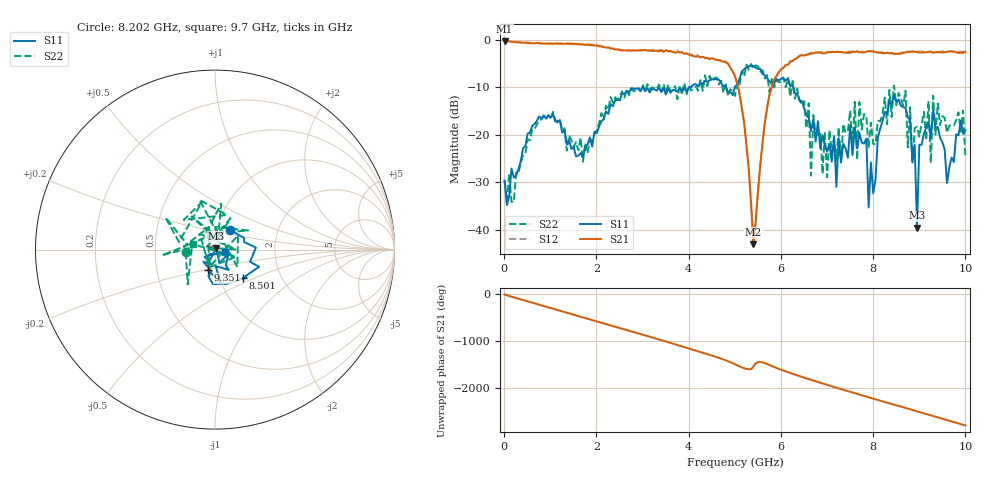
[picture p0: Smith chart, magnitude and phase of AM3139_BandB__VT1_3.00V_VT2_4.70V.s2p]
! Date/Time: Tue, Nov 13, 2018 5:00 PM
! Network Analyzer: Agilent Technologies E8364B Rev: A.07.50.67
! Sweep from 0.010 to 10.000 GHz, 201 Points, Sweep Type: LIN
! Power Supply: 3.001 V, 0.000 A
# Hz S DB R 50
!freq MagS11 AngS11 MagS21 AngS21 MagS12 AngS12 MagS22 AngS22
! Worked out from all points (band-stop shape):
!   201 points, 10 MHz to 10 GHz, reference 50 ohm
!   highest |S21| = -0.27 dB at 10 MHz (marker M1); lowest = -42.9 dB at 5.405 GHz (marker M2)
!   |S21| within 3 dB of the highest: start of sweep to 4.047 GHz; 6.523 GHz to end of sweep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
!   lowest |S11| = -39.5 dB at 8.951 GHz (marker M3), VSWR 1.02, Z = 50.7 + j0.819 ohm
!   |S11| at or under -10 dB: start of sweep to 2.997 GHz; 3.016 GHz to 4.008 GHz (991.9 MHz wide, 28.2 % of centre); 6.27 GHz to end of sweep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
!   |S22| runs from -34.1 to -5.1 dB; largest |S21 - S12| = 0.032
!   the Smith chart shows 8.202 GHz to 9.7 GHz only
!   S11 on the Smith chart (normalised r, x): 8.202 GHz: 1.15, +0.26; 8.501 GHz: 1.29, -0.43; 9.351 GHz: 0.90, -0.21; 9.7 GHz: 1.12, -0.03
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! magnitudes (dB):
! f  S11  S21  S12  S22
! 10 MHz  -29.6  -0.3  -0.2  -29.5
! 1.059 GHz  -15.6  -0.9  -0.8  -15.2
! 1.708 GHz  -24.7  -1.0  -0.9  -25.6
! 3.357 GHz  -10.2  -2.5  -2.2  -9.4
! 5.005 GHz  -9.8  -7.7  -7.7  -11.8
! 5.405 GHz  -5.6  -42.9  -43.4  -6.2
! 5.804 GHz  -8.8  -9.9  -9.9  -8.2
! 6.603 GHz  -16.4  -3.1  -3.0  -13.4
! 6.653 GHz  -19.1  -2.9  -2.7  -28.6
! 6.703 GHz  -16.7  -2.9  -2.7  -15.8
! 7.003 GHz  -23.5  -2.7  -2.6  -28.9
! 7.852 GHz  -20.8  -2.5  -2.4  -16.0
! 7.902 GHz  -35.2  -2.4  -2.4  -22.7
! 8.202 GHz  -17.2  -2.8  -2.6  -15.7
! 8.352 GHz  -12.8  -2.8  -2.9  -10.6
! 8.501 GHz  -13.1  -3.0  -2.8  -13.8
! 8.901 GHz  -22.1  -2.5  -2.6  -18.6
! 8.951 GHz  -39.5  -2.6  -2.5  -18.3
! 9.001 GHz  -22.1  -2.7  -2.5  -20.4
! 9.351 GHz  -18.5  -2.6  -2.6  -19.9
! 9.7 GHz  -24.8  -2.4  -2.5  -17.8
! 10 GHz  -19.0  -2.5  -2.5  -24.7
